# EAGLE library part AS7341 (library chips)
11-Channel Spectral Sensor Frontend
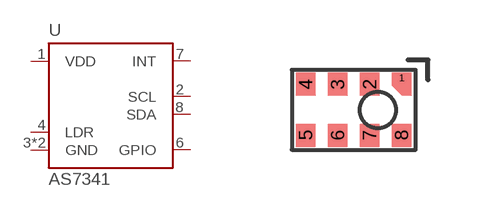
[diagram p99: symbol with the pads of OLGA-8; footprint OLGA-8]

Designator prefix U

## AS7341 (DIGIKEY: AS7341-DLGTCT-ND; MANUFACTURER: AMS; MPN: AS7341)  [OLGA-8]
1  VDD
2  SCL
3  GND
4  LDR
5  GND
6  GPIO
7  INT
8  SDA

## Footprint OLGA-8 (pad centres in mm)
8-PIN smd package for AS7341 color spectrum sensor
smd 0.25 x 0.25: 1 0.591,0.8
smd 0.488 x 0.575: 2 -0.209,0.638; 3 -1.009,0.638; 4 -1.809,0.638; 5 -1.809,-0.638; 6 -1.009,-0.638; 7 -0.209,-0.638; 8 0.591,-0.638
